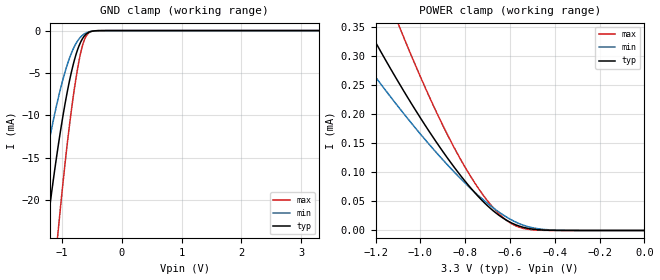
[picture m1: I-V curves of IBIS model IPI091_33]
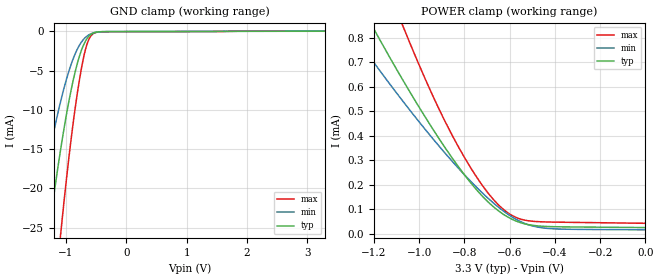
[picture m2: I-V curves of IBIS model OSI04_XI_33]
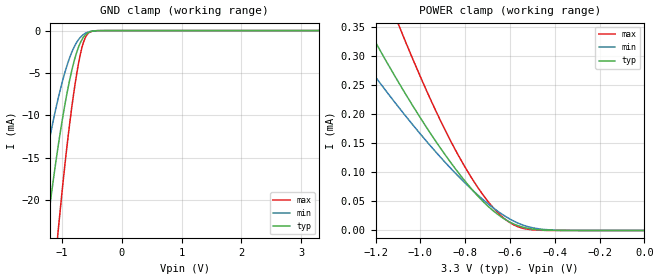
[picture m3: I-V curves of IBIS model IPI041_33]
| TEXAS INSTRUMENTS INCORPORATED
| Connectivity Solutions Group
| IBIS Model of TL16C2752FN_33V
| 2752FN_33V
| This file contains package information for the following:
|  FN 44-pin (PLCC) package as [Component] 2752FN_33V
| This device can be powered at the following Vccs:
|  3.3 volt Vcc
| This file provides unique models under the [Model Selector] for each Vcc.
| For operation at a specific Vcc, select the appropriate model after each
| [Model Selector] keyword.
[IBIS Ver]   3.2
[Comment char]  |_char
[File Name]   2752FN_33v.ibs
[File Rev]   1 | a
[Date]   August 8, 2006
[Source]   Data created from TI-SPICE simulations at TI-CONN.
[Notes]   The following is an IBIS list for the 2752FN_33V.
   Please contact s-ly@ti.com with questions and
   comments concerning CONN IBIS models.
[Disclaimer] Property of Texas Instruments Incorporated.  Unauthorized
   reproduction and/or distribution is strictly prohibited.
   This product is protected under copyright law.
   Created  2003, (C) Copyright  2003, Texas Instruments
   Incorporated, All Rights Reserved
   UNLESS THERE IS A SIGNED, WRITTEN AGREEMENT TO THE
   CONTRARY, TEXAS INSTRUMENTS (TI) IS PROVIDING THE IBIS
   MODELS  AND WITHOUT ANY WARRANTY, EXPRESSED OR
   IMPLIED.  TI assumes no liability for:
   1) the accuracy of the IBIS models provided to your
   company;
   2) the proper functioning of these IBIS Models in your
   design or for any resulting applications; or
   3) infringement of patents, copyrights or intellectual
   property rights resulting from your use of these IBIS
   models.
   TI provides IBIS Models as a service to our customers.
   You and your company shall not distribute, sell or give
   these models to anyone else without prior written
   permission from TI.
   TI reserves the right to make changes to our products or
   to discontinue any semiconductor product or service
   without notice, and advises our customers to obtain the
   latest version of relevant information to verify, before
   placing orders, that the information being relied on is
   current.
   Please be aware that your receipt and use of the IBIS
   information provided shall serve as acceptance of these
   terms and conditions.  If you do not accept these terms,
   you should return or destroy the IBIS models and any
   other accompanying information immediately.
| Component 2752_33V_PLCC 44-pin FN
[Component]   2752FN_33V
[Manufacturer]   Texas Instruments, Inc.
[Package]
|   typ   min   max
R_pkg   0.27365   0.25611   0.29119
L_pkg   3.46300n   3.21362n   3.71238n
C_pkg   0.17921p   0.17274p   0.18568p
1   TXRDYA   OPJ430   0.26610   3.35203n   0.17924p
2   D0   IPI04_OPJ43   0.25619   3.21362n   0.17274p
3   D1   IPI04_OPJ43   0.25703   3.22554n   0.17463p
4   D2   IPI04_OPJ43   0.26223   3.29838n   0.17902p
5   D3   IPI04_OPJ43   0.27188   3.43361n   0.18430p
6   D4   IPI04_OPJ43   0.28894   3.67285n   0.18405p
7   D5   IPI04_OPJ43   0.29092   3.70140n   0.18430p
8   D6   IPI04_OPJ43   0.27461   3.47357n   0.18401p
9   D7   IPI04_OPJ43   0.26580   3.35093n   0.17962p
10   A0   IPI041   0.26009   3.27164n   0.17623p
11   XTAL1   OSI04_XI   0.25816   3.24536n   0.17654p
12   GND   GND   0.26003   3.27223n   0.17871p
13   XTAL2   OSI04   0.25717   3.23295n   0.17470p
14   A1   IPI041   0.25762   3.23991n   0.17442p
15   A2   IPI041   0.26293   3.31463n   0.17955p
16   CHSEL   IPI041   0.27233   3.44671n   0.18401p
17   INTB   OPJ430   0.28853   3.67422n   0.18341p
18   CS   IPI041   0.28949   3.68860n   0.18516p
19   MFB   OPJ430   0.27189   3.44239n   0.18490p
20   IOW   IPI041   0.26222   3.30743n   0.17946p
21   RESET   IPI091   0.25694   3.23374n   0.17512p
22   GND   GND   0.25611   3.22234n   0.17417p
23   RTSB   OPJ430   0.25935   3.26764n   0.17611p
24   IOR   IPI041   0.25721   3.23771n   0.17415p
25   RXB   IPI041   0.25866   3.25783n   0.17500p
26   TXB   OPJ430   0.26418   3.33468n   0.18007p
27   DTRB   OPJ430   0.27430   3.47611n   0.18568p
28   CTSB   IPI041   0.29119   3.71238n   0.18515p
29   DSRB   IPI041   0.28780   3.66395n   0.18436p
30   CDB   IPI041   0.27039   3.41949n   0.18453p
31   RIB   IPI041   0.26088   3.28595n   0.17884p
32   TXRDYB   OPJ430   0.25629   3.22120n   0.17377p
33   VCC   POWER   0.25641   3.22223n   0.17297p
34   INTA   OPJ430   0.26011   3.27330n   0.17537p
35   MFA   OPJ430   0.25811   3.24463n   0.17410p
36   RTSA   OPJ430   0.25981   3.26771n   0.17557p
37   DTRA   OPJ430   0.26533   3.34432n   0.18028p
38   TXA   OPJ430   0.27534   3.48380n   0.18514p
39   RXA   IPI041   0.29078   3.69955n   0.18357p
40   CTSA   IPI041   0.28869   3.66932n   0.18288p
41   DSRA   IPI041   0.27269   3.44483n   0.18404p
42   CDA   IPI041   0.26282   3.30662n   0.17820p
43   RIA   IPI041   0.25821   3.24196n   0.17391p
44   VCC   POWER   0.25690   3.22349n   0.17422p
| Model IPI091
[Model Selector]   IPI091
IPI091_33   3.3 volt Vcc
| Model OSI04_XI
[Model Selector]   OSI04_XI
OSI04_XI_33   3.3 volt Vcc
| Model IPI041
[Model Selector]   IPI041
IPI041_33   3.3 volt Vcc
| Model IPI04_OPJ43
[Model Selector]   IPI04_OPJ43
IPI04_OPJ43_33   3.3 volt Vcc
| Model OPJ430
[Model Selector]   OPJ430
OPJ430_33   3.3 volt Vcc
| Model OSI04
[Model Selector]   OSI04
OSI04_33   3.3 volt Vcc
| Models and submodels in the file (6): IPI091_33 (Input), OSI04_XI_33 (Input), IPI041_33 (Input), IPI04_OPJ43_33 (I/O), OPJ430_33 (3-state), OSI04_33 (3-state)
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[Model]   IPI091_33
Model_type  Input
Vinl = 0
Vinh = 3.3
| variable   typ   min   max
C_comp   1.07pF   0.95pF   1.20pF
[Temperature Range]   40   125   -40
| Ambient temperature   25   110   -40
[Voltage range]   3.3   3   3.6
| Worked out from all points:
|   GND clamp passes 1 mA (typ) near -0.66 V on its own axis
|   POWER clamp passes 1 mA (typ) near -2.03 V on its own axis
[GND Clamp]
| IPI091_33
|   Voltage   I(typ)   I(min)   I(max)
-3.3V     -184.1mA   -131.7mA   -253.5mA
-1.485V   -37.43mA   -23.94mA   -59.12mA
-1.28V    -24.78mA   -15.34mA   -40.66mA
-1.25V    -23.07mA   -14.2mA    -38.11mA
-1.075V   -13.97mA   -8.224mA   -24.19mA
-1.06V    -13.26mA   -7.774mA   -23.08mA
-940mV    -8.152mA   -4.58mA    -14.87mA
-805mV    -3.718mA   -2.005mA   -7.28mA
-700mV    -1.488mA   -825uA     -2.909mA
-600mV    -421.4uA   -273uA     -659.6uA
-400mV    -8.531uA   -12.92uA   -6.748uA
3.3V      251.6pA    69.15nA    65.83pA
[POWER Clamp]
| IPI091_33
|   Voltage   I(typ)   I(min)   I(max)
-3.3V     2.289mA    1.713mA    3.253mA
-1.35V    432uA      344.6uA    613.8uA
-1.225V   341.4uA    277.2uA    481uA
-1.11V    263.3uA    218.6uA    366.4uA
-1.075V   240.6uA    201.5uA    333.1uA
-930mV    152.9uA    134.7uA    205.1uA
-805mV    87.01uA    83.43uA    112uA
-700mV    42.42uA    46.59uA    50.87uA
-620mV    18.66uA    24.18uA    18.85uA
-540mV    5.375uA    9.01uA     3.55uA
-445mV    638.3nA    1.643uA    187.2nA
-47.99fV  251.6pA    2.2nA      73.1pA
[Model]   OSI04_XI_33
Model_type  Input
Vinl = 0
Vinh = 3.3
| variable   typ   min   max
C_comp   1.85pF   1.15pF   2.42pF
[Temperature Range]   40   125   -40
| Ambient temperature   25   110   -40
[Voltage range]   3.3   3   3.6
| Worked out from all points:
|   GND clamp passes 1 mA (typ) near -0.66 V on its own axis
|   POWER clamp passes 1 mA (typ) near -1.30 V on its own axis
[GND Clamp]
| OSI04_XI_33
|   Voltage   I(typ)   I(min)   I(max)
-3.3V     -187.4mA   -133.6mA   -258.6mA
-1.52V    -40.73mA   -26.12mA   -63.96mA
-1.48V    -38.05mA   -24.28mA   -60.12mA
-1.275V   -25.2mA    -15.59mA   -41.32mA
-1.095V   -15.43mA   -9.17mA    -26.46mA
-1.07V    -14.21mA   -8.387mA   -24.55mA
-935mV    -8.294mA   -4.704mA   -15.09mA
-800mV    -3.791mA   -2.104mA   -7.36mA
-695mV    -1.529mA   -912.1uA   -2.917mA
-600mV    -479.4uA   -361uA     -744.5uA
-390mV    -35.35uA   -32.95uA   -52.71uA
3.3V      25.17uA    17.8uA     39.06uA
[POWER Clamp]
| OSI04_XI_33
|   Voltage   I(typ)   I(min)   I(max)
-3.3V     5.294mA    3.984mA    7.572mA
-1.3V     1.007mA    827.6uA    1.402mA
-1.195V   827.7uA    692.7uA    1.14mA
-1.075V   632.4uA    545.1uA    855.7uA
-1.04V    577.7uA    503.5uA    776.7uA
-915mV    392.6uA    361.2uA    514.8uA
-815mV    259.4uA    256uA      336.3uA
-720mV    152.9uA    166.1uA    196.6uA
-625mV    77.8uA     91.06uA    97.45uA
-555mV    46.18uA    50.98uA    60.77uA
-455mV    30.55uA    24.01uA    48.59uA
-47.99fV  25.17uA    16.02uA    42.63uA
[Model]   IPI041_33
Model_type  Input
Vinl = 0
Vinh = 3.3
| variable   typ   min   max
C_comp   1.08pF   0.95pF   1.21pF
[Temperature Range]   40   125   -40
| Ambient temperature   25   110   -40
[Voltage range]   3.3   3   3.6
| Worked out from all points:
|   GND clamp passes 1 mA (typ) near -0.66 V on its own axis
|   POWER clamp passes 1 mA (typ) near -2.03 V on its own axis
[GND Clamp]
| IPI041_33
|   Voltage   I(typ)   I(min)   I(max)
-3.3V     -184.1mA   -131.7mA   -253.5mA
-1.485V   -37.43mA   -23.94mA   -59.12mA
-1.28V    -24.78mA   -15.34mA   -40.66mA
-1.25V    -23.07mA   -14.2mA    -38.11mA
-1.075V   -13.97mA   -8.224mA   -24.19mA
-1.06V    -13.26mA   -7.774mA   -23.08mA
-940mV    -8.152mA   -4.58mA    -14.87mA
-805mV    -3.718mA   -2.005mA   -7.28mA
-700mV    -1.488mA   -825uA     -2.909mA
-600mV    -421.4uA   -273uA     -659.6uA
-400mV    -8.531uA   -12.92uA   -6.748uA
3.3V      251.6pA    69.15nA    65.83pA
[POWER Clamp]
| IPI041_33
|   Voltage   I(typ)   I(min)   I(max)
-3.3V     2.289mA    1.713mA    3.253mA
-1.35V    432uA      344.6uA    613.8uA
-1.225V   341.4uA    277.2uA    481uA
-1.11V    263.3uA    218.6uA    366.4uA
-1.075V   240.6uA    201.5uA    333.1uA
-930mV    152.9uA    134.7uA    205.1uA
-805mV    87.01uA    83.43uA    112uA
-700mV    42.42uA    46.59uA    50.87uA
-620mV    18.66uA    24.18uA    18.85uA
-540mV    5.375uA    9.01uA     3.55uA
-445mV    638.3nA    1.643uA    187.2nA
-47.99fV  251.6pA    2.2nA      73.1pA
